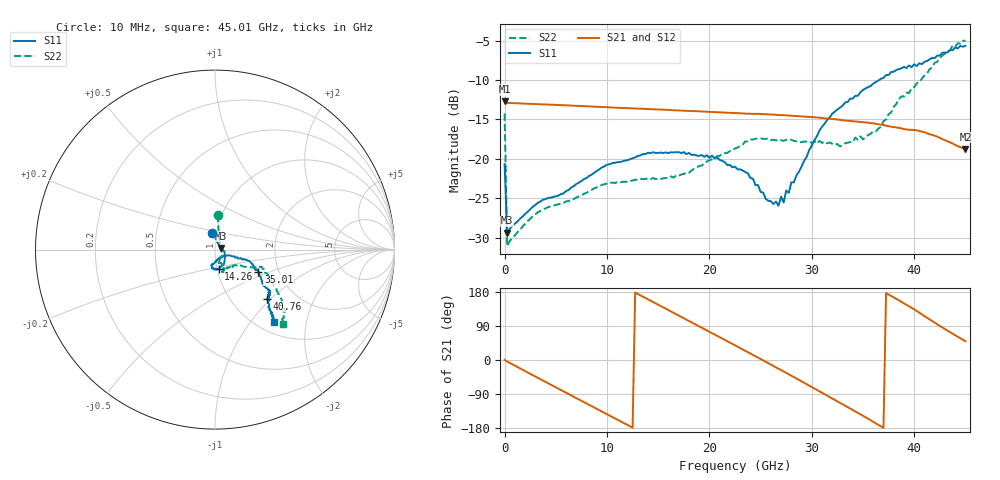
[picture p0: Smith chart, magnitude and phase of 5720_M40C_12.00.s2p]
! Device:  ADRF5720
! Description: 0.5dB LSB GaAs MMIC 6-bit Digital Attenuator
! Frequency:  0.000009 -  40 GHz
! Ports:
!	RF1	= Port 1
!	RF2	= Port 2
! Vdd:  3.3 Volt
! Vss:  -3.3 Volt
! Control:  0/3.3 Volt
! State:  12.00 dB attenuation
! Data:  The device was measured using G-S-G Probes on a matrix board.
!  Data was collected using an calibrated 4 port network analyzer.
!  The reference plane for this measurement is at the launchers.
! Note:  Analog Devices supplies this data as a sample of measured data
!  for this product.  Your particular data for this product may vary.
!  Data was taken at -40 degrees C.
!  Analog Devices reserves the right to change this data at anytime.
# GHZ S DB R 45.0
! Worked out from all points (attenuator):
!   181 points, 10 MHz to 45.01 GHz, reference 45 ohm
!   highest |S21| = -12.72 dB at 10 MHz (marker M1); lowest = -18.7 dB at 45.01 GHz (marker M2)
!   lowest |S11| = -29.4 dB at 260 MHz (marker M3), VSWR 1.07, Z = 48.1 + j0.817 ohm
!   |S11| at or under -10 dB: start of sweep to 36.59 GHz
!   |S22| runs from -31.1 to -5.0 dB; largest |S21 - S12| = 0.00091
!   S11 on the Smith chart (normalised r, x): 10 MHz: 0.95, +0.17; 14.26 GHz: 1.02, -0.22; 35.01 GHz: 1.57, -0.43; 40.76 GHz: 1.45, -0.95; 45.01 GHz: 1.18, -1.31
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0.01  -20.66 101.7  -12.72 0.1  -12.74 0.1  -14.26 85.6
0.26  -29.35 14.4  -12.90 -3.9  -12.92 -4.0  -31.06 15.4
3.26  -25.55 -12.5  -13.07 -47.2  -13.09 -47.3  -26.75 -27.7
7.76  -22.56 -43.0  -13.31 -111.2  -13.33 -111.2  -24.43 -61.5
11.26  -20.39 -62.1  -13.53 -160.8  -13.55 -160.9  -22.99 -74.0
14.26  -19.26 -78.9  -13.70 156.6  -13.71 156.5  -22.57 -76.8
15.26  -19.20 -83.3  -13.75 142.3  -13.77 142.2  -22.54 -75.5
19.01  -19.62 -96.7  -13.97 88.9  -14.00 88.8  -20.91 -64.2
22.76  -21.32 -102.9  -14.20 35.1  -14.23 35.0  -18.57 -65.8
24.01  -22.42 -93.5  -14.28 17.2  -14.31 17.1  -17.52 -67.1
26.76  -25.94 -52.0  -14.45 -23.1  -14.47 -23.2  -17.56 -69.5
27.01  -24.77 -47.2  -14.46 -26.6  -14.48 -26.8  -17.63 -71.5
27.26  -25.53 -43.9  -14.47 -30.4  -14.49 -30.5  -17.71 -70.1
27.51  -24.01 -37.7  -14.47 -34.0  -14.49 -34.2  -17.58 -71.3
27.76  -24.31 -34.0  -14.51 -37.8  -14.54 -38.0  -17.64 -69.8
30.26  -17.66 -18.9  -14.72 -75.2  -14.75 -75.3  -17.75 -69.0
32.01  -14.26 -18.7  -14.95 -101.5  -14.97 -101.7  -18.08 -60.6
35.01  -11.27 -27.6  -15.35 -147.2  -15.37 -147.4  -17.54 -41.8
37.76  -8.99 -37.0  -15.92 169.1  -15.94 168.8  -14.10 -29.0
40.76  -7.98 -43.3  -16.54 120.4  -16.58 120.2  -9.82 -24.9
43.76  -6.24 -48.5  -18.04 69.3  -18.07 69.2  -5.64 -41.4
45.01  -5.68 -51.1  -18.73 49.6  -18.77 49.5  -4.99 -47.5
